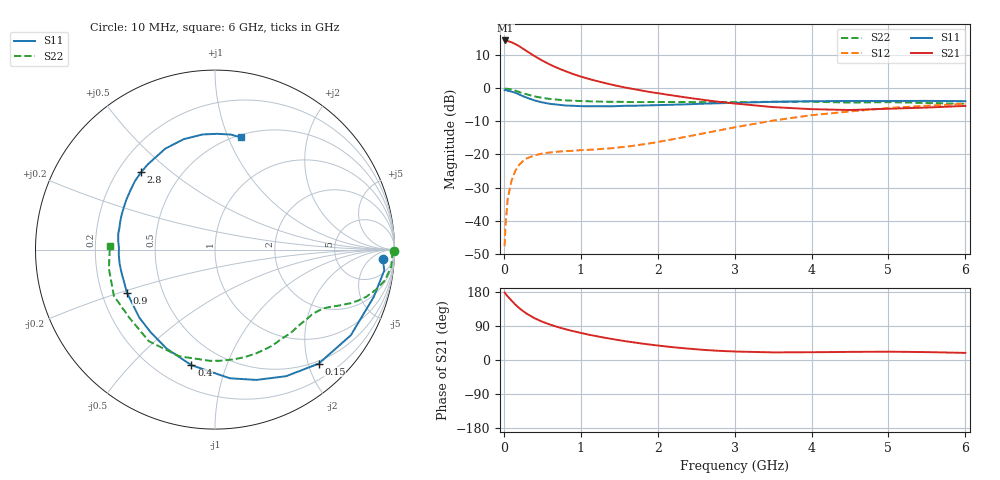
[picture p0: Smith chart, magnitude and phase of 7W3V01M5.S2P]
! Infineon Technologies  Discrete & RF Semiconductors
! BFS17W
! Si NPN RF Bipolar Junction Transistor in SOT323
! VCE = 3 V  IC = 1.5 mA
! Common Emitter S-Parameters:  August  1999
# GHz  S  MA  R  50
!  f  S11  S21  S12  S22
! GHz  MAG  ANG  MAG  ANG  MAG  ANG  MAG  ANG
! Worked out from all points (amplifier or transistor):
!   36 points, 10 MHz to 6 GHz, reference 50 ohm
!   highest |S21| = 14.5 dB at 20 MHz (marker M1)
!   |S21| within 3 dB of that: start of sweep to 282.1 MHz
!   unconditionally stable (mu >= 1): 902.3 MHz to end of sweep
!   at 250 MHz: K = 0.31, MSG = 17.0 dB, |S12| = -22.0 dB
!   at 1.4 GHz: K = 1.32, MAG = 6.2 dB, |S12| = -18.1 dB
!   at 6 GHz: K = 1.10, MAG = -2.3 dB, |S12| = -4.7 dB
!   S11 on the Smith chart (normalised r, x): 10 MHz: 18, -15; 150 MHz: 0.45, -2.18; 400 MHz: 0.34, -0.76; 900 MHz: 0.31, -0.21; 2.8 GHz: 0.30, +0.40; 6 GHz: 0.52, +1.11
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0.01  0.9363 -3.2  5.258 178.3  0.0041 85.3  1 -0.6
0.02  0.9503 -7.0  5.312 175.2  0.0079 88.7  0.988 -2.0
0.05  0.9228 -16.6  5.198 167.9  0.0212 80.3  0.987 -5.3
0.1  0.8948 -32.2  4.986 156.9  0.0403 72.2  0.9636 -10.1
0.15  0.8587 -47.7  4.682 146.1  0.0568 63.8  0.9228 -14.1
0.2  0.8089 -60.7  4.351 137.0  0.07 58.2  0.8831 -17.3
0.25  0.7618 -72.4  3.976 129.0  0.0797 52.1  0.8435 -19.8
0.3  0.7217 -83.4  3.646 121.9  0.0875 48.1  0.8115 -21.6
0.4  0.6572 -101.5  3.081 110.2  0.0971 42.0  0.756 -24.4
0.5  0.614 -116.0  2.635 101.1  0.1034 38.4  0.719 -26.3
0.6  0.5835 -128.0  2.291 93.5  0.1073 36.3  0.6924 -28.1
0.7  0.5671 -138.0  2.03 87.0  0.1104 35.5  0.6747 -29.9
0.9  0.546 -154.0  1.65 76.2  0.1136 35.8  0.6499 -33.9
1.1  0.5364 -166.5  1.396 66.9  0.1177 38.0  0.6381 -38.4
1.4  0.5353 179.0  1.14 55.7  0.1241 43.1  0.6282 -45.8
1.6  0.5465 170.4  1.017 49.0  0.1317 47.1  0.6224 -51.2
2.2  0.5666 150.9  0.779 33.7  0.1703 58.1  0.622 -68.4
2.8  0.5961 133.7  0.626 24.2  0.232 62.2  0.6199 -86.9
3.5  0.6269 116.3  0.521 20.1  0.3258 59.6  0.627 -108.6
4.5  0.6453 96.2  0.471 21.4  0.4476 47.7  0.6099 -141.5
5.5  0.647 82.3  0.513 20.8  0.5465 35.0  0.6007 -169.8
6  0.6413 77.1  0.543 18.8  0.5847 28.9  0.5856 177.8
